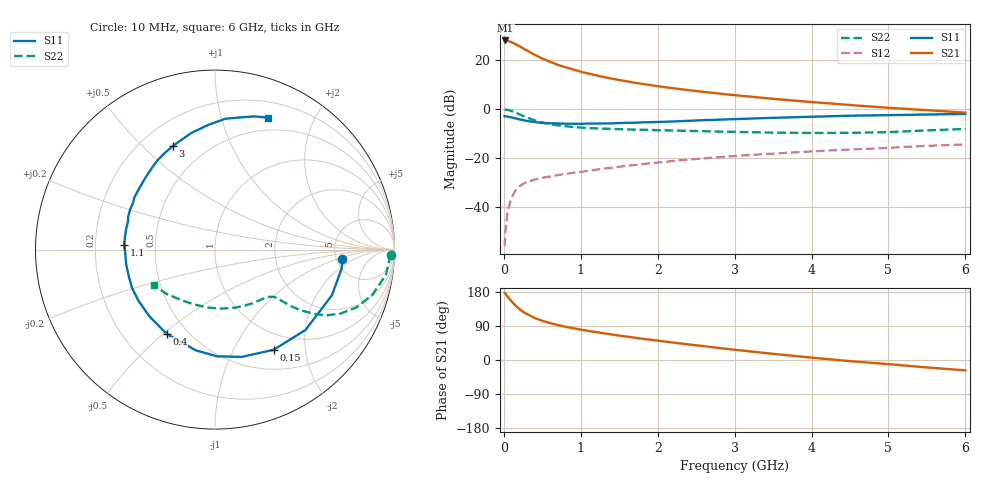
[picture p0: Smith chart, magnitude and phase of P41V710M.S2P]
! SIEMENS Small Signal Semiconductors
! BFP182
! Si NPN RF Bipolar Junction Transistor in SOT143
! VCE = 1.75 V  IC = 10 mA
! Common Emitter S-Parameters:  March  1996
# GHz  S  MA  R  50
!  f  S11  S21  S12  S22
! GHz  MAG  ANG  MAG  ANG  MAG  ANG  MAG  ANG
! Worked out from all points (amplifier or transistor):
!   36 points, 10 MHz to 6 GHz, reference 50 ohm
!   highest |S21| = 28.0 dB at 20 MHz (marker M1)
!   |S21| within 3 dB of that: start of sweep to 237.9 MHz
!   unconditionally stable (mu >= 1): 1.095 GHz to 5.448 GHz
!   at 250 MHz: K = 0.34, MSG = 27.7 dB, |S12| = -30.6 dB
!   at 1.4 GHz: K = 1.12, MAG = 16.1 dB, |S12| = -24.0 dB
!   at 6 GHz: K = 0.95, MSG = 6.5 dB, |S12| = -14.4 dB
!   S11 on the Smith chart (normalised r, x): 10 MHz: 5.65, -1.25; 150 MHz: 0.76, -1.46; 400 MHz: 0.39, -0.51; 1.1 GHz: 0.33, +0.02; 3 GHz: 0.33, +0.62; 6 GHz: 0.36, +1.42
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0.01  0.7117 -4.4  24.9 177.5  0.0016 88.7  0.9795 -1.6
0.02  0.7133 -8.6  25.01 175.1  0.0032 85.7  0.973 -3.4
0.05  0.6994 -21.4  24.64 166.9  0.0083 83.4  0.9628 -8.4
0.1  0.6742 -41.6  23.02 154.8  0.0156 69.7  0.9121 -16.0
0.15  0.6467 -59.6  21.18 144.1  0.0218 63.1  0.852 -22.2
0.2  0.6164 -75.8  19.27 134.8  0.0264 58.2  0.7847 -27.0
0.25  0.5948 -88.9  17.24 127.3  0.0296 53.0  0.7236 -30.4
0.3  0.5715 -100.8  15.6 121.4  0.0326 50.4  0.6711 -32.5
0.4  0.5413 -119.9  12.81 111.0  0.0365 46.8  0.5885 -35.2
0.5  0.5211 -134.8  10.7 103.4  0.0398 43.9  0.5313 -36.6
0.6  0.5128 -146.3  9.232 97.4  0.0421 42.9  0.4932 -37.1
0.7  0.5091 -155.4  7.994 92.3  0.045 43.3  0.4666 -37.6
0.9  0.5016 -170.5  6.403 84.0  0.0501 43.6  0.4307 -38.3
1.1  0.5064 177.2  5.291 76.5  0.0555 44.0  0.4102 -39.9
1.3  0.5081 167.6  4.48 70.4  0.0609 44.2  0.3977 -41.6
1.6  0.5235 154.4  3.669 61.6  0.0697 44.3  0.3842 -45.3
2.2  0.5579 133.8  2.653 46.0  0.0871 42.9  0.3656 -54.8
3  0.6228 112.3  1.92 27.1  0.1103 38.1  0.3421 -71.3
3.5  0.6626 101.6  1.613 16.2  0.1235 34.5  0.3307 -83.5
4.5  0.7313 85.5  1.207 -3.0  0.1497 27.1  0.3269 -110.8
5.5  0.7737 73.6  0.947 -19.6  0.1782 19.7  0.3665 -137.7
6  0.7924 68.1  0.846 -27.4  0.1897 14.8  0.393 -150.3
